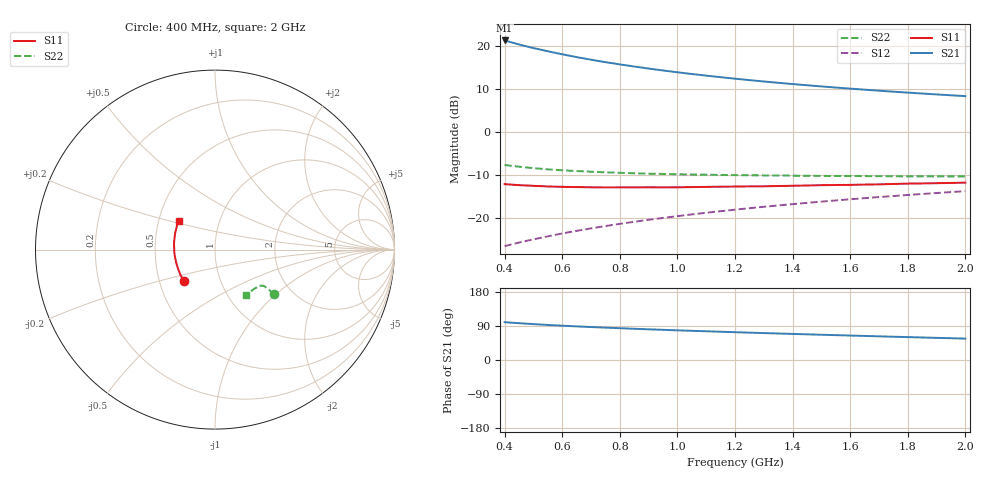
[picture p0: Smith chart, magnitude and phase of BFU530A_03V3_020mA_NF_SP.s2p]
! Filename:  P:\Prog\Test\Noise\ATS_data\Testdata_Net\06 Compressed Noise after Statistics\BFU530A_APG2013_33_A05_03p3V_020mA_NF_CM01_D.sf
! Date/Time: Tue 16/Apr/2013 15:11:06
! BFU530A_APG2013_33_A05_03p3V_1to25mA_NF_CM01_Bias7_R.sf
! Noise Parameter Data File
! BFU530A_APG2013_33_A05_03p3V_1to25mA_NF_CM01
! Date/time: Fri Apr 12 14:21:19 2013
! VAR V_out= 3.300000
! VAR I_out= 20.000000
! VAR V_in= 0.851100
! VAR I_in= 0.225150
! Device data file deembeded for feedlines and parallel
! Original file: \06 Compressed Noise after Statistics\BFU530A_APG2013_33_A05_03p3V_020mA_NF_CM01_R.sf
! Feed-files: PR017V01_150413_Feed1.s2p, PR017V01_150413_Feed2.s2p
! Parallel-file: PR017V01_150413_Par.s2p
# MHz S MA R 50
!  Freq-MHz  S11-mag  S11-arg  S21-mag  S21-arg  S12-mag  S12-arg  S22-mag  S22-arg
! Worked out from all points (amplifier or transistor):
!   37 points, 400 MHz to 2 GHz, reference 50 ohm
!   highest |S21| = 21.3 dB at 400 MHz (marker M1)
!   |S21| within 3 dB of that: start of sweep to 584.3 MHz
!   unconditionally stable (mu >= 1): 886.6 MHz to 1.889 GHz
!   at 500 MHz: K = 0.94, MSG = 22.2 dB, |S12| = -25.0 dB
!   at 1.1 GHz: K = 1.01, MAG = 15.4 dB, |S12| = -18.8 dB
!   at 2 GHz: K = 1.00, MSG = 11.0 dB, |S12| = -13.8 dB
!   lowest NFmin = 1.02 dB at 433 MHz
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400  0.2471 -134.4  11.59 99.9  0.04695 71.0  0.4133 -37.2
420  0.2448 -136.9  11.09 98.7  0.04886 71.2  0.405 -37.1
440  0.2421 -139.5  10.64 97.6  0.05077 71.4  0.3979 -37.0
480  0.2382 -144.1  9.823 95.7  0.05452 71.8  0.3853 -36.8
500  0.2364 -146.4  9.46 94.7  0.05641 71.9  0.38 -36.8
550  0.2323 -151.6  8.678 92.5  0.06108 72.3  0.3671 -36.5
600  0.23 -156.0  7.999 90.5  0.06596 72.6  0.3583 -36.4
650  0.2285 -160.0  7.423 88.7  0.07079 72.8  0.3511 -36.5
700  0.2272 -163.7  6.925 87.0  0.07561 72.9  0.3448 -36.6
750  0.2265 -167.3  6.487 85.4  0.08048 73.0  0.3392 -36.8
800  0.2267 -170.4  6.106 83.9  0.08534 73.0  0.3351 -37.1
850  0.2268 -173.6  5.767 82.4  0.09023 73.0  0.3306 -37.5
900  0.2273 -176.5  5.463 81.0  0.09514 73.0  0.3272 -37.8
950  0.227 -179.2  5.19 79.6  0.1 72.9  0.3248 -38.3
1050  0.2283 175.8  4.721 77.0  0.1099 72.7  0.32 -39.3
1150  0.2308 171.2  4.334 74.6  0.1198 72.3  0.316 -40.5
1200  0.2318 169.1  4.165 73.4  0.1248 72.1  0.3149 -41.2
1350  0.2352 163.0  3.731 69.9  0.1397 71.3  0.3116 -43.4
1500  0.2405 157.5  3.384 66.7  0.1547 70.5  0.3081 -45.8
1600  0.2424 154.1  3.191 64.5  0.1648 69.8  0.3073 -47.6
1750  0.2484 149.3  2.941 61.4  0.1798 68.8  0.3052 -50.3
2000  0.2575 142.1  2.61 56.5  0.205 66.9  0.304 -55.4
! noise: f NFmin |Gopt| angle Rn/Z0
400  1.056  0.2664  -168.2  0.0813
460  1.046  0.2696  -166.9  0.0758
600  1.164  0.2434  -161  0.0905
800  1.113  0.3035  -156.8  0.0758
1000  1.115  0.3121  -151.7  0.0799
1200  1.158  0.3269  -146.5  0.0859
1400  1.221  0.335  -143.4  0.0879
1600  1.211  0.3677  -135.6  0.0981
1800  1.24  0.387  -130.5  0.1008
2000  1.24  0.3896  -127  0.1169
